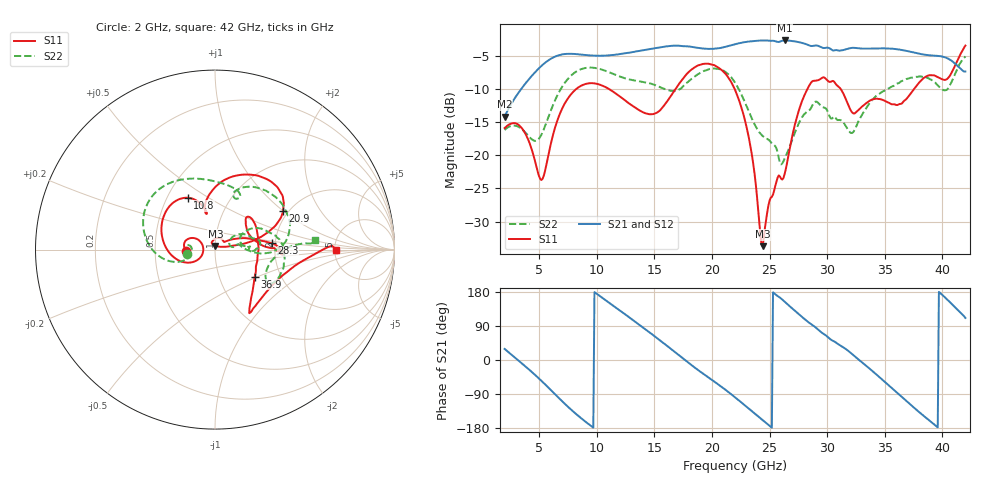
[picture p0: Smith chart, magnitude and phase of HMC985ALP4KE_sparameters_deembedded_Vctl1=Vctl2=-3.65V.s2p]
!s2p File: Measurements: S11, S21, S12, S22
# GHz S dB R 50.0
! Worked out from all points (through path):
!   401 points, 2 GHz to 42 GHz, reference 50 ohm
!   highest |S21| = -2.66 dB at 26.3 GHz (marker M1); lowest = -14.2 dB at 2 GHz (marker M2)
!   lowest |S11| = -33.7 dB at 24.4 GHz (marker M3), VSWR 1.04, Z = 50.2 + j2.06 ohm
!   |S11| at or under -10 dB: start of sweep to 8.207 GHz; 21.97 GHz to 28.28 GHz (6.312 GHz wide, 25.1 % of centre); 31.17 GHz to 37.54 GHz (6.367 GHz wide, 18.5 % of centre)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
!   |S22| runs from -21.4 to -5.1 dB; largest |S21 - S12| = 0.00059
!   S11 on the Smith chart (normalised r, x): 2 GHz: 0.72, -0.01; 10.8 GHz: 0.63, +0.41; 20.9 GHz: 1.88, +1.00; 28.3 GHz: 1.92, +0.15; 36.9 GHz: 1.48, -0.48; 42 GHz: 5.12, -0.00
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2  -15.89 -176.6  -14.18 29.2  -14.18 29.2  -16.17 -171.9
3.5  -15.91 157.9  -9.85 -9.1  -9.85 -9.1  -16.05 171.3
5.2  -23.73 -179.6  -6.50 -55.0  -6.50 -55.0  -16.87 -166.5
6.8  -13.71 -162.3  -4.85 -103.1  -4.85 -103.1  -10.22 -172.5
8.7  -9.45 149.5  -4.80 -155.0  -4.80 -155.0  -6.96 150.2
10.8  -9.74 117.6  -4.94 157.0  -4.95 157.0  -7.27 115.8
13.3  -12.75 103.7  -4.36 101.8  -4.35 101.8  -8.70 80.1
15.4  -13.35 104.7  -3.73 53.9  -3.73 53.9  -9.63 64.8
17.9  -7.56 76.4  -3.55 -5.8  -3.55 -5.8  -8.94 69.5
20.9  -7.20 29.6  -3.73 -72.4  -3.74 -72.4  -7.11 18.6
22  -10.10 18.2  -3.23 -98.4  -3.23 -98.3  -9.02 0.9
23.3  -18.25 11.7  -2.81 -130.8  -2.80 -130.7  -13.80 -3.3
24.4  -33.71 83.4  -2.66 -158.4  -2.66 -158.4  -17.08 10.1
26.3  -22.86 38.1  -2.66 154.1  -2.66 154.1  -20.52 30.1
28.3  -9.94 6.3  -3.30 101.4  -3.30 101.4  -13.35 17.9
28.7  -8.83 0.5  -3.50 93.0  -3.50 93.0  -12.51 15.3
32.4  -13.65 29.9  -3.78 9.5  -3.78 9.5  -16.10 26.1
33.9  -11.58 43.7  -3.88 -28.4  -3.88 -28.4  -11.65 27.6
35.4  -12.10 14.3  -3.88 -68.5  -3.87 -68.5  -9.85 16.7
36.9  -11.45 -34.2  -4.24 -109.0  -4.24 -109.0  -8.47 4.0
39.6  -8.19 -56.4  -4.99 -177.7  -4.99 -177.7  -9.45 -31.6
42  -3.44 -0.0  -7.34 110.9  -7.34 110.9  -5.07 5.4
